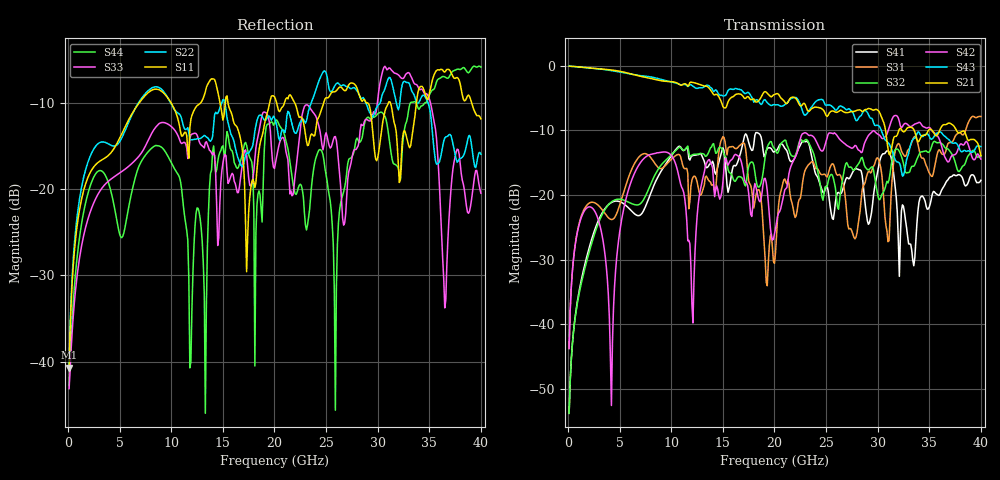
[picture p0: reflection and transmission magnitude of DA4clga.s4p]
! ADC12DJ3200QML-SP
! 196-pin ZMX package
! CLGA Ceramic Package without columns (ceramic land grid array)
! Texas Instruments 4/21/2021
! Single-ended  S-parameters
! PORT#  PORT_NAME  NET_NAME
! PORT1:  DAxN.DIEBUMP DAxN
! PORT2:  DAxN.BGA  DAxN
! PORT3:  DAxP.DIEBUMP DAxP
! PORT4:  DAxP.BGA  DAxP
! Touchstone Ver. 1.0
! Number of ports is 4
# Hz	S	MA	R	50.000000
! SCATTERING PARAMETERS  :
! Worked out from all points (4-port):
!   400 points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, 100 MHz to 40 GHz, reference 50 ohm
!   strongest paths, dB at 100 MHz, 10.1 GHz, 20.1 GHz, 30.1 GHz, 40 GHz:
!     S21: -0.1, -2.5, -4.4, -7.0, -13.9
!     S43: -0.1, -2.5, -6.0, -9.3, -12.5
!     S42: -43.7, -14.1, -25.2, -10.7, -14.4
!     S32: -53.7, -13.6, -13.1, -20.6, -13.9
!     S31: -43.7, -14.3, -28.9, -14.5, -7.8
!     S41: -53.7, -13.7, -13.1, -15.5, -17.7
!   lowest |S11| = -40.7 dB at 100 MHz (marker M1), VSWR 1.02, Z = 50.6 - j0.714 ohm
!   |S11| at or under -10 dB: start of sweep to 6.866 GHz; 10 GHz to 12.82 GHz (2.813 GHz wide, 24.7 % of centre); 15.5 GHz to 19.52 GHz (4.025 GHz wide, 23 % of centre)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
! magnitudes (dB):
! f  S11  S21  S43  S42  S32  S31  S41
! 100 MHz  -40.7  -0.1  -0.1  -43.7  -53.7  -43.7  -53.7
! 10.7 GHz  -12.1  -2.8  -2.8  -16.8  -12.7  -13.7  -12.5
! 13.3 GHz  -8.7  -3.1  -3.1  -15.5  -14.0  -17.2  -15.4
! 14.1 GHz  -7.2  -4.5  -4.0  -18.0  -12.0  -18.6  -15.2
! 24.5 GHz  -10.9  -6.6  -5.2  -13.1  -19.1  -16.8  -18.7
! 25.9 GHz  -8.6  -7.2  -6.8  -10.5  -18.9  -16.2  -21.2
! 40 GHz  -11.8  -13.9  -12.5  -14.4  -13.9  -7.8  -17.7
